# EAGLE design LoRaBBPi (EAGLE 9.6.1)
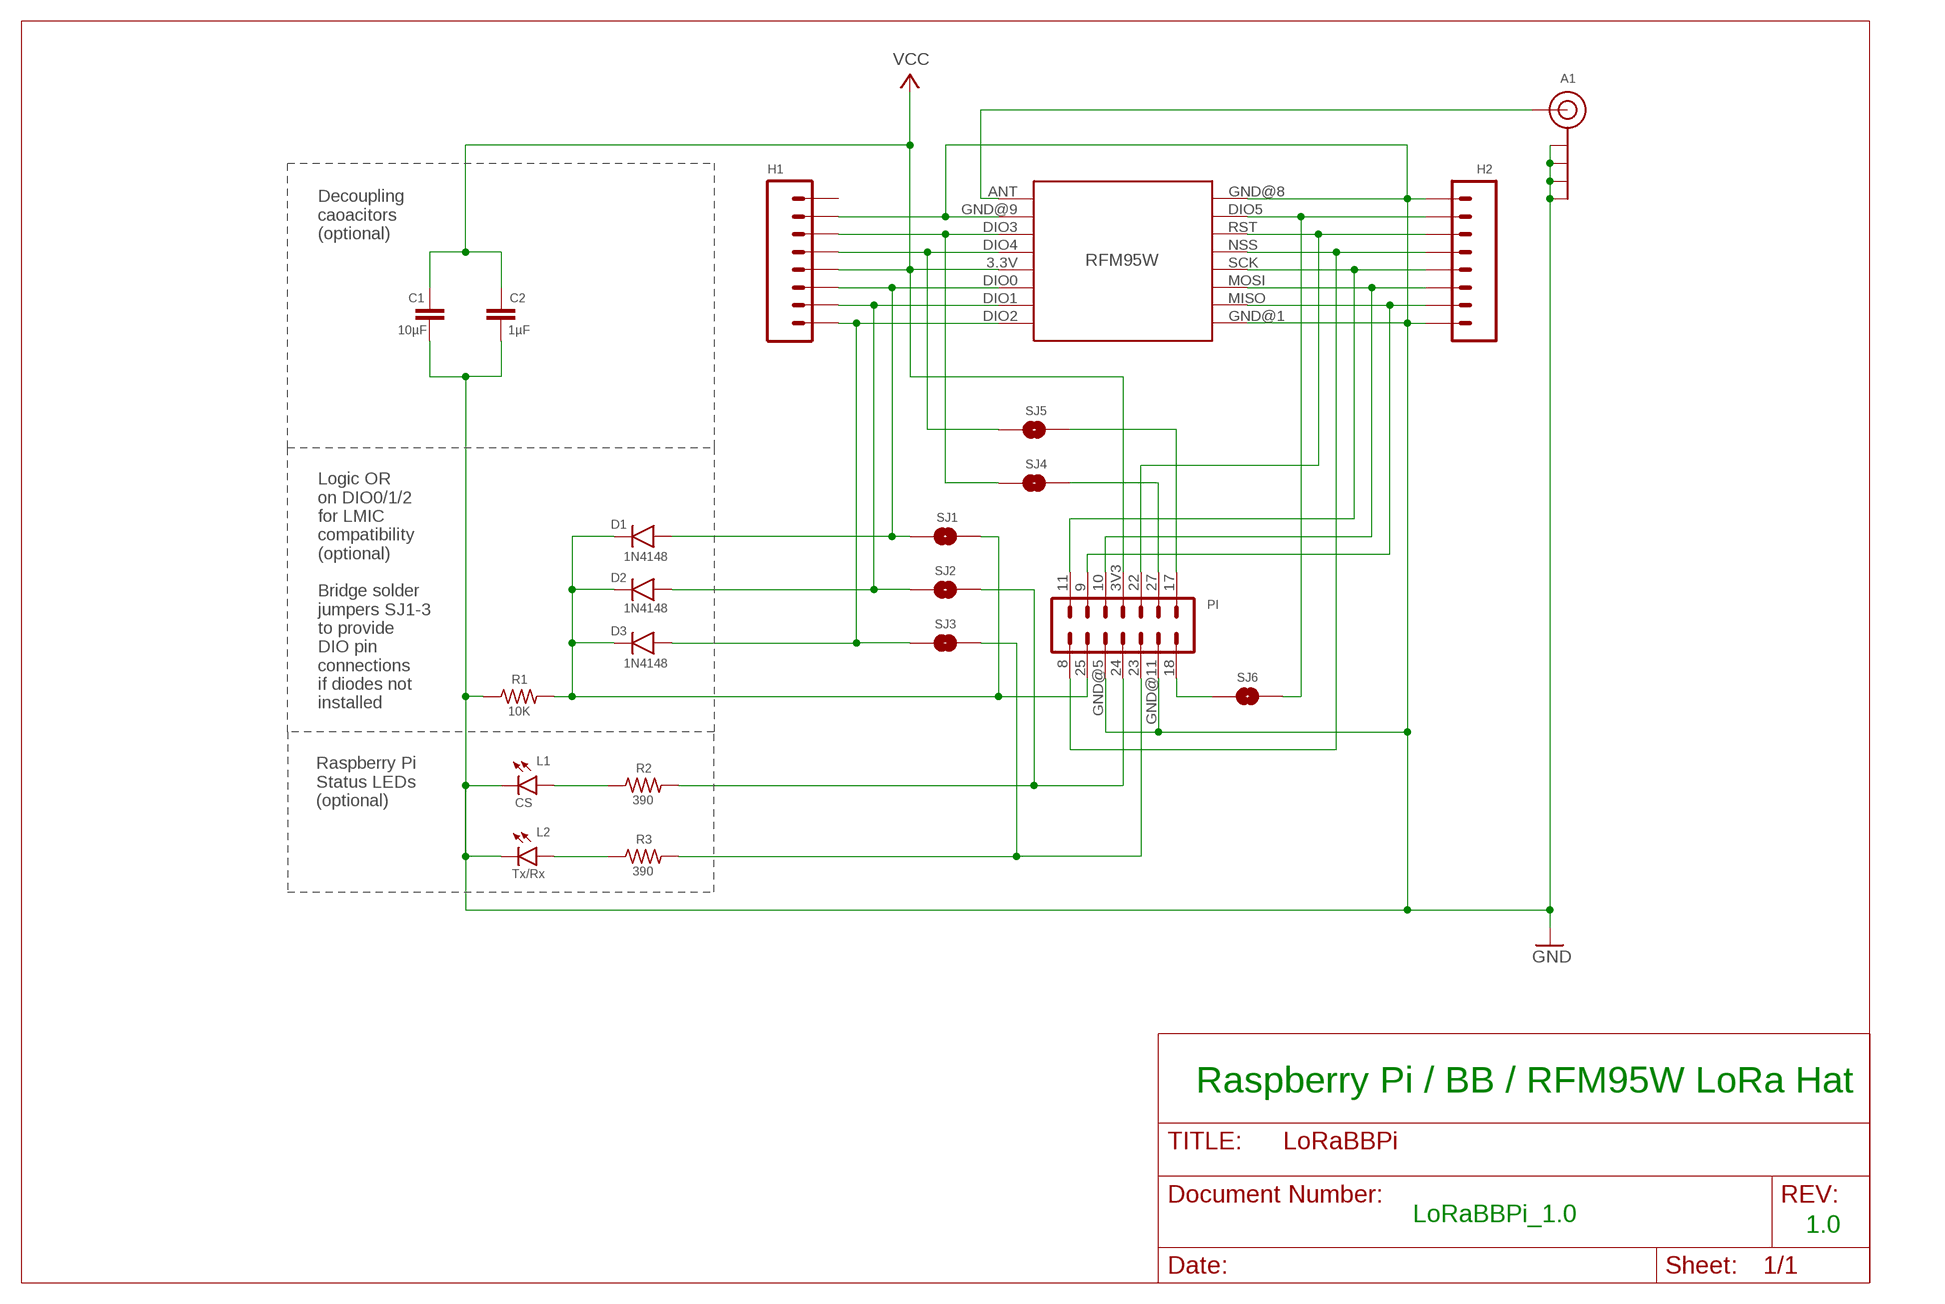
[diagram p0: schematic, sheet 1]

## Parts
A1  U.FL-SMA-EDGE-COMBO  [U.FL-SMA-EDGE-COMBO]
C1  10µF  CAPACITOR  [C0805]
C2  1µF  CAPACITOR  [C0805]
D1  1N4148  1N4148SMD  [SOD-123]
D2  1N4148  1N4148SMD  [SOD-123]
D3  1N4148  1N4148SMD  [SOD-123]
H1  1X8-PIN-HEADER  [1X8]
H2  1X8-PIN-HEADER  [1X8]
L1  CS  LEDCHIP-LED0805  [CHIP-LED0805]
L2  Tx/Rx  LEDCHIP-LED0805  [CHIP-LED0805]
PI  2X7-PIN-HEADER  [2X7]
R1  10K  R-US_R0805  [R0805]
R2  390  R-US_R0805  [R0805]
R3  390  R-US_R0805  [R0805]
RFM95W  RFM95W-LORA  [RFM95W-LORA]
SJ1  SJ  [SJ]
SJ2  SJ  [SJ]
SJ3  SJ  [SJ]
SJ4  SJ  [SJ]
SJ5  SJ  [SJ]
SJ6  SJ  [SJ]

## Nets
GND: A1.GND@1A(GND) A1.GND@1B(GND) A1.GND@2A(GND) A1.GND@2B(GND) C1.2 C2.2 H1.2 H2.1 H2.8 L1.C L2.C PI.GND@5(GND) PI.GND@11(GND) R1.1 RFM95W.GND@1(GND.1) RFM95W.GND@8(GND.2) RFM95W.GND@9(GND.3)
N$1: L2.A R3.1
N$2: L1.A R2.1
N$3: PI.18 SJ6.1
N$4: H2.4 PI.8 RFM95W.NSS
N$5: PI.23 R3.2 SJ3.2
N$6: PI.24 R2.2 SJ2.2
N$7: D1.2 H1.6 RFM95W.DIO0 SJ1.1
N$8: H1.4 RFM95W.DIO4 SJ5.1
N$9: H1.3 RFM95W.DIO3 SJ4.1
N$10: D1.1 D2.1 D3.1 PI.25 R1.2 SJ1.2
N$11: A1.SIG RFM95W.ANT
N$12: D2.2 H1.7 RFM95W.DIO1 SJ2.1
N$13: H2.3 PI.22 RFM95W.RST
N$14: D3.2 H1.8 RFM95W.DIO2 SJ3.1
N$15: H2.5 PI.11 RFM95W.SCK
N$16: H2.6 PI.10 RFM95W.MOSI
N$17: H2.7 PI.9 RFM95W.MISO
N$18: PI.27 SJ4.2
N$19: PI.17 SJ5.2
N$20: H2.2 RFM95W.DIO5 SJ6.2
VCC: C1.1 C2.1 H1.5 PI.3V3 RFM95W.3.3V
Unconnected: H1.1

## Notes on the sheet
- Decoupling
  caoacitors
  (optional)
- Logic OR
  on DIO0/1/2
  for LMIC
  compatibility
  (optional)
  
  Bridge solder
  jumpers SJ1-3
  to provide
  DIO pin
  connections
  if diodes not
  installed
- Raspberry Pi
  Status LEDs
  (optional)
- Raspberry Pi / BB / RFM95W LoRa Hat
- LoRaBBPi_1.0
- 1.0

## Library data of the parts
A1 = digitalconcepts:U.FL-SMA-EDGE-COMBO: Combination u.FL & SMA edge mount antenna
C1 C2 = digitalconcepts:CAPACITOR: 0805 Capacitor
D1-D3 = digitalconcepts:1N4148: 1N4148 SOD-123 Signal Diode
H1 H2 = digitalconcepts:1X8-PIN-HEADER: Single Row 8-Pin Header
L1 L2 = led:LED: LED
PI = digitalconcepts:2X7-PIN-HEADER: Double Row 14-Pin Header
R1-R3 = digitalconcepts:R-US_: RESISTOR, American symbol; SPICEPREFIX: R
RFM95W = digitalconcepts:RFM95W-LORA: RFM95W LoRa Wireless Transceiver
SJ1-SJ6 = digitalconcepts:SJ: Solder Jumper

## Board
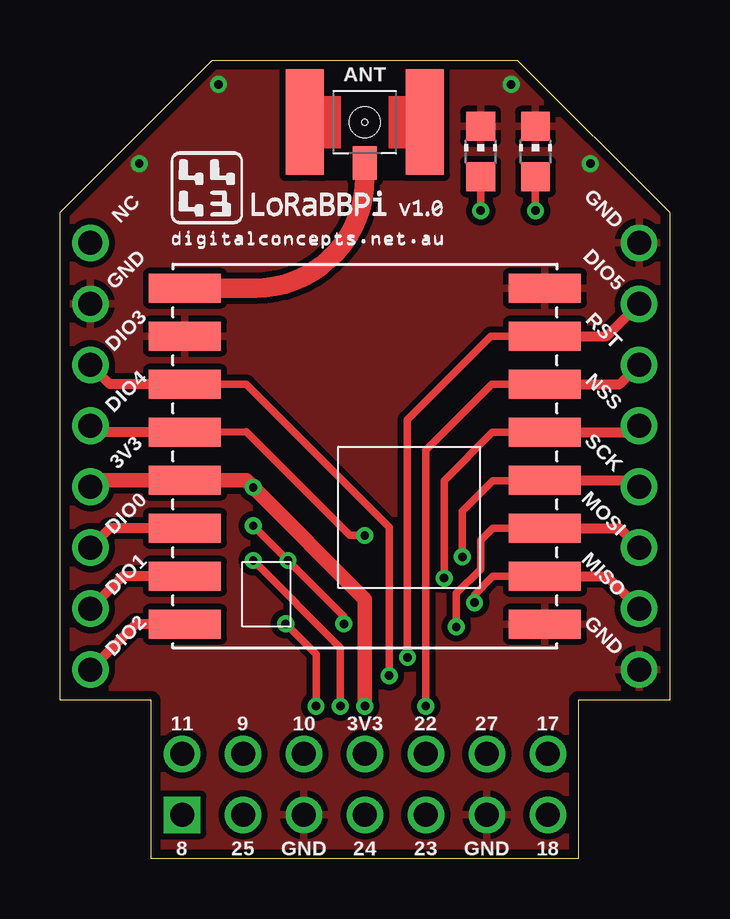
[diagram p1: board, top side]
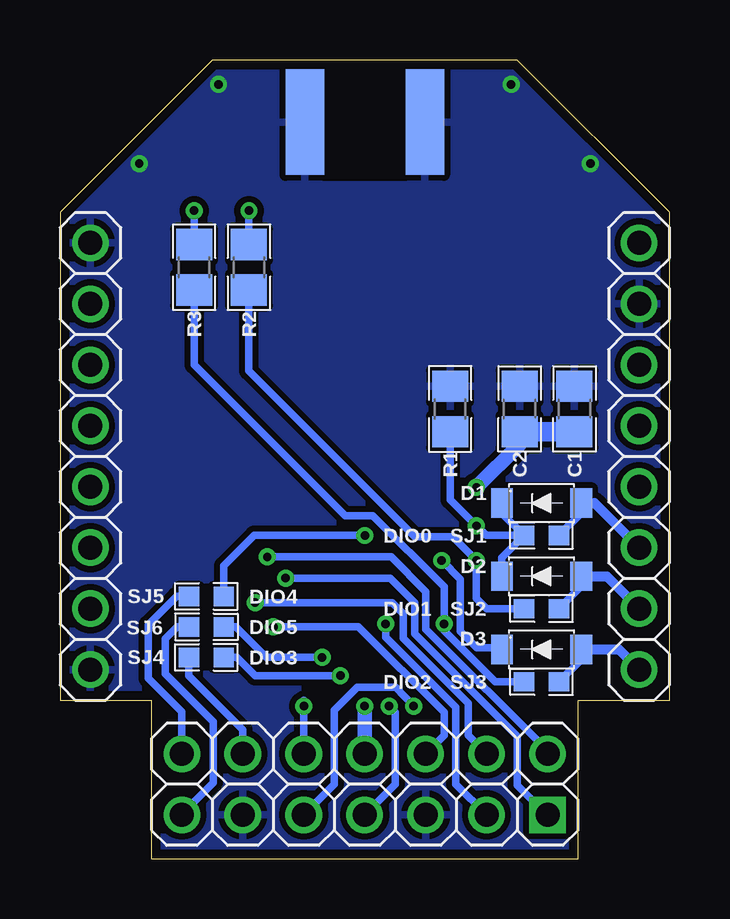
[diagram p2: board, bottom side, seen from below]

Size 25.4 x 33.27 mm. Coordinates in mm from the lower left corner, seen from the top.
Outline: 0,6.6 0,26.92 6.35,33.27 19.05,33.27 25.4,26.92 25.4,6.6 21.59,6.6 21.59,0 3.81,0 3.81,6.6 0,6.6
Copper layers (1*16): Top 0.0356mm / dielectric 1.5011mm / Bottom 0.0356mm
Design rules "PCBs_io": minimum track width 6mil, minimum drill 13mil, track to track 6mil, track to pad 6mil, pad to pad 6mil, via to via 6mil, smd to smd 6mil, copper to edge 15mil, drill to drill 6mil, minimum pad ring 7mil, minimum via ring 7mil, stop-mask expansion 3mil, vias tented up to drill 0mil, thermal gap 10mil

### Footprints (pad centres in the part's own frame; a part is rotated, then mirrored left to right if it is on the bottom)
U.FL-SMA-EDGE-COMBO = smd 1.6 x 4.4: GND@1A -2.5,0; GND@2A 2.5,0 | smd 1.6 x 4.4 bottom: GND@1B -2.5,0; GND@2B 2.5,0 | smd 1 x 1.4: SIG 0,-1.7
C0805 = smd 1.3 x 1.5: 1 -0.95,0; 2 0.95,0
SOD-123 = smd 0.91 x 1.22: 1 1.65,0; 2 -1.65,0
1X8 = drill 1 pad 1.524: 1 0,0; 2 2.54,0; 3 5.08,0; 4 7.62,0; 5 10.16,0; 6 12.7,0; 7 15.24,0; 8 17.78,0
CHIP-LED0805 = smd 1.2 x 1.2: A 0,-1.05; C 0,1.05
2X7 = drill 1 pad 1.524: 3V3 7.62,2.54; 9 2.54,2.54; 10 5.08,2.54; 11 0,2.54; 17 15.24,2.54; 18 15.24,0; 22 10.16,2.54; 23 10.16,0; 24 7.62,0; 25 2.54,0; 27 12.7,2.54; GND@5 5.08,0; GND@11 12.7,0 | drill 1 pad 1.524 square: 8 0,0
R0805 = smd 1.3 x 1.5: 1 -0.95,0; 2 0.95,0
RFM95W-LORA = smd 3 x 1.2: 3.3V 7.5,1; ANT 7.5,-7; DIO0 7.5,3; DIO1 7.5,5; DIO2 7.5,7; DIO3 7.5,-3; DIO4 7.5,-1; DIO5 -7.5,-5; GND@1 -7.5,7; GND@8 -7.5,-7; GND@9 7.5,-5; MISO -7.5,5; MOSI -7.5,3; NSS -7.5,-1; RST -7.5,-3; SCK -7.5,1
SJ = smd 0.85 x 0.8: 1 -0.725,0; 2 0.725,0

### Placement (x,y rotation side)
A1  12.7,30.68 0 top
C1  3.96,18.74 90 bottom
C2  6.25,18.74 90 bottom
D1  5.33,14.81 180 bottom
D2  5.33,11.76 180 bottom
D3  5.33,8.71 180 bottom
H1  1.27,25.65 270 top
H2  24.13,25.65 270 top
L1  17.53,29.46 0 top
L2  19.81,29.46 0 top
PI  5.09,1.82 0 top
R1  9.14,18.74 270 bottom
R2  17.53,24.64 270 bottom
R3  19.81,24.64 270 bottom
RFM95W  12.7,16.76 180 top
SJ1  5.33,13.46 180 bottom
SJ2  5.33,10.41 180 bottom
SJ3  5.33,7.37 180 bottom
SJ4  19.3,8.38 180 bottom
SJ5  19.3,10.92 180 bottom
SJ6  19.3,9.65 0 bottom

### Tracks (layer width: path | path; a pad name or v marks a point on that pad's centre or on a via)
GND  (via drill 0.35)
  other vias: 3.3,28.96 6.6,32.26 18.8,32.26 22.1,28.96
  pour Top (isolate 0.254): 6.35,33.27 19.05,33.27 25.4,26.92 25.4,6.6 21.59,6.6 21.59,0 3.81,0 3.81,6.6 0,6.6 0,26.92
  pour Bottom (isolate 0.254): 6.35,33.27 19.05,33.27 25.4,26.92 25.4,6.6 21.59,6.6 21.59,0 3.81,0 3.81,6.6 0,6.6 0,26.92
N$1  (via drill 0.35)
  Top 0.305: L2.A v19.81,27
  Bottom 0.305: R3.1 v19.81,27
N$2  (via drill 0.35)
  Top 0.305: L1.A v17.53,27
  Bottom 0.305: R2.1 v17.53,27
N$3
  Bottom 0.305: PI.18 20.32,1.84 19,3.16 19,5.69 21.01,7.7 21.01,9.16 20.52,9.65 SJ6.1
N$4  (via drill 0.35)
  Top 0.305: v16,11.68 16,15.75 18.02,17.76 RFM95W.NSS
  Top 0.406: H2.4 23.86,17.76 RFM95W.NSS
  Bottom 0.305: v16,11.68 11.65,11.68 10.63,10.67 10.63,9.37 6.35,5.09 6.35,3.05 5.12,1.82 PI.8
N$5  (via drill 0.35)
  Top 0.305: v9.4,9.78 10.67,8.51 v10.67,6.35
  Bottom 0.305: SJ3.2 7.27,7.37 9.4,9.49 v9.4,9.78 9.4,11.32 12.36,14.28 13.52,14.28 19.81,20.57 R3.2 | PI.23 13.97,3.1 13.97,6.17 13.01,7.13 11.4,7.13 v10.67,6.35
N$6  (via drill 0.35)
  Top 0.305: v8.05,12.42 11.68,8.79 v11.68,6.35
  Bottom 0.305: SJ2.2 7.62,10.41 8.05,10.85 v8.05,12.42 9.04,13.41 10.61,13.41 17.53,20.32 R2.2 | PI.24 11.43,3.1 11.43,6.1 v11.68,6.35
N$7
  Top 0.406: H1.6 2.08,13.76 RFM95W.DIO0
  Bottom 0.305: D1.2 3.68,14.39 SJ1.1
  Bottom 0.406: D1.2 3.13,14.81 H1.6
N$8  (via drill 0.35)
  Top 0.305: RFM95W.DIO4 7.76,17.78 12.07,13.46 v12.7,13.46
  Top 0.406: H1.4 1.54,17.76 RFM95W.DIO4
  Bottom 0.305: v12.7,13.46 17.32,13.46 18.58,12.2 SJ5.1
N$9  (via drill 0.35)
  Top 0.305: v13.72,7.62 13.72,13.8 7.76,19.76 RFM95W.DIO3
  Top 0.406: H1.3 2.08,19.76 RFM95W.DIO3
  Bottom 0.305: SJ4.1 18.03,8.38 17.27,7.62 v13.72,7.62
N$10  (via drill 0.35)
  Top 0.305: v8.05,13.87 v9.5,12.42 11.83,10.09 v11.83,9.78
  Bottom 0.152: D3.1 7.05,8.78
  Bottom 0.305: v11.83,9.78 11.83,9.22 8.9,6.29 8.9,3.1 PI.25 | SJ1.2 6.98,12.54 D2.1 | D1.1 6.98,14.39 SJ1.2 | 7.05,8.78 8.03,8.78 8.71,9.46 8.71,11.64 v9.5,12.42 | R1.2 9.14,14.96 v8.05,13.87 7.64,13.46 SJ1.2
N$11
  Top 0.813: A1.SIG 12.7,28.35 arc-90 8.11,23.76 RFM95W.ANT
N$12
  Top 0.406: H1.7 2.62,11.76 RFM95W.DIO1
  Bottom 0.305: D2.2 3.68,11.34 SJ2.1
  Bottom 0.406: H1.7 2.62,11.76 D2.2
N$13  (via drill 0.35)
  Top 0.305: v15.24,6.35 15.24,17.02 17.99,19.76 RFM95W.RST
  Top 0.406: H2.3 23.32,19.76 RFM95W.RST
  Bottom 0.305: v15.24,6.35 15.24,6.6 PI.22
N$14
  Top 0.406: H1.8 3.16,9.76 RFM95W.DIO2
  Bottom 0.305: D3.2 3.68,8.29 SJ3.1
  Bottom 0.406: D3.2 2.11,8.71 H1.8
N$15  (via drill 0.35)
  Top 0.305: v16.76,12.57 16.76,14.48 18.03,15.75 20.18,15.75 RFM95W.SCK
  Top 0.406: H2.5 23.86,15.76 RFM95W.SCK
  Bottom 0.305: PI.11 5.09,4.49 10.15,9.56 10.15,11.12 11.6,12.57 v16.76,12.57
N$16  (via drill 0.35)
  Top 0.305: RFM95W.MOSI 18.03,13.76 17.53,13.26 17.53,12.06 16.51,11.05 v16.51,9.65
  Top 0.406: RFM95W.MOSI 23.32,13.76 H2.6
  Bottom 0.305: PI.10 9.4,5.13 9.4,6.1 12.97,9.65 v16.51,9.65
N$17  (via drill 0.35)
  Top 0.305: RFM95W.MISO 18.03,11.76 17.27,11 v17.27,10.67
  Top 0.406: H2.7 22.78,11.76 RFM95W.MISO
  Bottom 0.305: v17.27,10.67 11.56,10.67 11.1,10.21 11.1,9.18 8.39,6.47 8.39,5.13 PI.9
N$18
  Bottom 0.305: PI.27 17.78,5.38 20.03,7.62 SJ4.2
N$19
  Bottom 0.305: PI.17 20.32,6.11 21.72,7.51 21.72,9.73 20.54,10.92 SJ5.2
N$20  (via drill 0.35)
  Top 0.305: RFM95W.DIO5 17.95,21.76 14.48,18.29 v14.48,8.38
  Top 0.406: H2.2 22.79,21.76 RFM95W.DIO5
  Bottom 0.305: SJ6.2 18.07,9.65 16.8,8.38 v14.48,8.38
VCC  (via drill 0.35)
  Top 0.305: 12.7,10.81 12.7,10.8
  Top 0.61: 12.7,10.8 v12.7,6.35 | H1.5 1.54,15.76 RFM95W.3.3V 7.76,15.76 v8.05,15.47 12.7,10.81
  Bottom 0.61: C2.1 6.25,17.27 v8.05,15.47 | PI.3V3 v12.7,6.35
  Bottom 0.813: C1.1 C2.1

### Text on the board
tPlace: ANT | NC | GND | GND | DIO5 | DIO3 | RST | DIO4 | NSS | 3V3 | SCK | DIO0 | MOSI | DIO1 | MISO | DIO2 | GND | 11 | 9 | 10 | 3V3 | 22 | 27 | 17 | 8 | 25 | GND | 24 | 23 | GND | 18
bPlace: DIO0 | DIO4 | DIO1 | DIO5 | DIO3 | DIO2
